| ORCA 4E IBIS file
[IBIS ver]   2.1
[File name]   t_all4e.ibs
[File Rev]   1.3
[Date]   07-29-2004
[Source]   Simulation
[Notes]   IBIS model for ORCA I/O
   These models are non-monotonic to more accurately reflect
   device function. The user should use appropriate IBIS
   simulation techniques.
[Disclaimer] The data in this model is derived from simulations using
   modeling information extracted from the target process. While
   a great deal of care has been taken to provide information
   that is accurate, this model is considered preliminary as it
   has not been verified by actual silicon measurement.Treat the
   data in this model as preliminary until actual silicon
   verification is performed.
[Copyright]   None
|   Component t_all4e
[Component]   t_all4e
[Manufacturer]   Lattice Semiconductor
[Package]
| variable   typ   min   max
| Package BA 352
R_pkg   0.3000   0.2600   0.3300
L_pkg   12.0000nH   10.0000nH   14.0000nH
C_pkg   2.0000pF   1.5000pF   2.5000pF
| Package BC432
|R_pkg   0.4100   0.3400   0.4700
|L_pkg   7.5000nH   6.5000nH   9.5000nH
|C_pkg   1.3000pF   1.1500pF   1.8000pF
|Package BM680
|R_pkg   0.3000   0.2600   0.3500
|L_pkg   7.0000nH   5.5000nH   9.5000nH
|C_pkg   0.8500pF   0.700pF   1.5000pF
[Pin]  signal_name   model_name   R_pin   L_pin   C_pin
101   OBLTTL6   OBLTTL6
102   IBLTTL   IBLTTL
103   OZLTTL6   OZLTTL6
104   BZLTTL6   BZLTTL6
105   IBLTTLPD   IBLTTLPD
106   OZLTTL6PD   OZLTTL6PD
107   BZLTTL6PD   BZLTTL6PD
108   IBLTTLPU   IBLTTLPU
109   OZLTTL6PU   OZLTTL6PU
110   BZLTTL6PU   BZLTTL6PU
111   OBLTTL12   OBLTTL12
112   OZLTTL12   OZLTTL12
113   BZLTTL12   BZLTTL12
114   OZLTTL12PD   OZLTTL12PD
115   BZLTTL12PD   BZLTTL12PD
116   OZLTTL12PU   OZLTTL12PU
117   BZLTTL12PU   BZLTTL12PU
118   OBLTTL24   OBLTTL24
119   OZLTTL24   OZLTTL24
120   BZLTTL24   BZLTTL24
121   OZLTTL24PD   OZLTTL24PD
122   BZLTTL24PD   BZLTTL24PD
123   OZLTTL24PU   OZLTTL24PU
124   BZLTTL24PU   BZLTTL24PU
125   OBCMOS186   OBCMOS186
126   IBCMOS18   IBCMOS18
127   OZCMOS186   OZCMOS186
128   BZCMOS186   BZCMOS186
129   IBCMOS18PD   IBCMOS18PD
130   OZCMOS186PD   OZCMOS186PD
131   BZCMOS186PD   BZCMOS186PD
132   IBCMOS18PU   IBCMOS18PU
133   OZCMOS186PU   OZCMOS186PU
134   BZCMOS186PU   BZCMOS186PU
135   OBCMOS1812   OBCMOS1812
136   OZCMOS1812   OZCMOS1812
137   BZCMOS1812   BZCMOS1812
138   OZCMOS1812PD   OZCMOS1812PD
139   BZCMOS1812PD   BZCMOS1812PD
140   OZCMOS1812PU   OZCMOS1812PU
141   BZCMOS1812PU   BZCMOS1812PU
142   OBCMOS1824   OBCMOS1824
143   OZCMOS1824   OZCMOS1824
144   BZCMOS1824   BZCMOS1824
145   OZCMOS1824PD   OZCMOS1824PD
146   BZCMOS1824PD   BZCMOS1824PD
147   OZCMOS1824PU   OZCMOS1824PU
148   BZCMOS1824PU   BZCMOS1824PU
149   OBCMOS26   OBCMOS26
150   IBCMOS2   IBCMOS2
151   OZCMOS26   OZCMOS26
152   BZCMOS26   BZCMOS26
153   IBCMOS2PD   IBCMOS2PD
154   OZCMOS26PD   OZCMOS26PD
155   BZCMOS26PD   BZCMOS26PD
156   IBCMOS2PU   IBCMOS2PU
157   OZCMOS26PU   OZCMOS26PU
158   BZCMOS26PU   BZCMOS26PU
159   OBCMOS212   OBCMOS212
160   OZCMOS212   OZCMOS212
161   BZCMOS212   BZCMOS212
162   OZCMOS212PD   OZCMOS212PD
163   BZCMOS212PD   BZCMOS212PD
164   OZCMOS212PU   OZCMOS212PU
165   BZCMOS212PU   BZCMOS212PU
166   OBCMOS224   OBCMOS224
167   OZCMOS224   OZCMOS224
168   BZCMOS224   BZCMOS224
169   OZCMOS224PD   OZCMOS224PD
170   BZCMOS224PD   BZCMOS224PD
171   OZCMOS224PU   OZCMOS224PU
172   BZCMOS224PU   BZCMOS224PU
173   OBGTL   OBGTL
174   IBGTL   IBGTL
175   OZGTL   OZGTL
176   BZGTL   BZGTL
177   OBGTLP   OBGTLP
178   IBGTLP   IBGTLP
179   OZGTLP   OZGTLP
180   BZGTLP   BZGTLP
181   OBHSTL   OBHSTL
182   IBHSTL   IBHSTL
183   OZHSTL   OZHSTL
184   BZHSTL   BZHSTL
185   OBPCI   OBPCI
186   IBPCI   IBPCI
187   OZPCI   OZPCI
188   BZPCI   BZPCI
189   OBPECL   OBPECL
190   IBPECL   IBPECL
191   OBSSTL3   OBSSTL3
192   IBSSTL3   IBSSTL3
193   OZSSTL3   OZSSTL3
194   BZSSTL3   BZSSTL3
195   OBSSTL2   OBSSTL2
196   IBSSTL2   IBSSTL2
197   OZSSTL2   OZSSTL2
198   BZSSTL2   BZSSTL2
203   OBLTTL6F   OBLTTL6F
204   OZLTTL6F   OZLTTL6F
205   BZLTTL6F   BZLTTL6F
206   OZLTTL6FPD   OZLTTL6FPD
207   BZLTTL6FPD   BZLTTL6FPD
208   OZLTTL6FPU   OZLTTL6FPU
209   BZLTTL6FPU   BZLTTL6FPU
210   OBLTTL12F   OBLTTL12F
211   OZLTTL12F   OZLTTL12F
212   BZLTTL12F   BZLTTL12F
213   OZLTTL12FPD   OZLTTL12FPD
214   BZLTTL12FPD   BZLTTL12FPD
215   OZLTTL12FPU   OZLTTL12FPU
216   BZLTTL12FPU   BZLTTL12FPU
217   OBLTTL24F   OBLTTL24F
218   OZLTTL24F   OZLTTL24F
219   BZLTTL24F   BZLTTL24F
220   OZLTTL24FPD   OZLTTL24FPD
221   BZLTTL24FPD   BZLTTL24FPD
222   OZLTTL24FPU   OZLTTL24FPU
223   BZLTTL24FPU   BZLTTL24FPU
224   OBCMOS186F   OBCMOS186F
225   OZCMOS186F   OZCMOS186F
226   BZCMOS186F   BZCMOS186F
227   OZCMOS186FPD   OZCMOS186FPD
228   BZCMOS186FPD   BZCMOS186FPD
229   OZCMOS186FPU   OZCMOS186FPU
230   BZCMOS186FPU   BZCMOS186FPU
231   OBCMOS1812F   OBCMOS1812F
232   OZCMOS1812F   OZCMOS1812F
233   BZCMOS1812F   BZCMOS1812F
234   OZCMOS1812FPD  OZCMOS1812FPD
235   BZCMOS1812FPD  BZCMOS1812FPD
236   OZCMOS1812FPU  OZCMOS1812FPU
237   BZCMOS1812FPU  BZCMOS1812FPU
238   OBCMOS1824F   OBCMOS1824F
239   OZCMOS1824F   OZCMOS1824F
240   BZCMOS1824F   BZCMOS1824F
241   OZCMOS1824FPD  OZCMOS1824FPD
242   BZCMOS1824FPD  BZCMOS1824FPD
243   OZCMOS1824FPU  OZCMOS1824FPU
244   BZCMOS1824FPU  BZCMOS1824FPU
245   OBCMOS26F   OBCMOS26F
246   OZCMOS26F   OZCMOS26F
247   BZCMOS26F   BZCMOS26F
248   OZCMOS26FPD   OZCMOS26FPD
249   BZCMOS26FPD   BZCMOS26FPD
250   OZCMOS26FPU   OZCMOS26FPU
251   BZCMOS26FPU   BZCMOS26FPU
252   OBCMOS212F   OBCMOS212F
253   OZCMOS212F   OZCMOS212F
254   BZCMOS212F   BZCMOS212F
255   OZCMOS212FPD   OZCMOS212FPD
256   BZCMOS212FPD   BZCMOS212FPD
257   OZCMOS212FPU   OZCMOS212FPU
258   BZCMOS212FPU   BZCMOS212FPU
259   OBCMOS224F   OBCMOS224F
260   OZCMOS224F   OZCMOS224F
261   BZCMOS224F   BZCMOS224F
262   OZCMOS224FPD   OZCMOS224FPD
263   BZCMOS224FPD   BZCMOS224FPD
264   OZCMOS224FPU   OZCMOS224FPU
265   BZCMOS224FPU   BZCMOS224FPU
266   OBHSTL18   OBHSTL18
267   IBHSTL18   IBHSTL18
268   OZHSTL18   OZHSTL18
269   BZHSTL18   BZHSTL18
301p   OBLVDSp   OBLVDS
301n   OBLVDSn   OBLVDS
302p   IBLVDSp   IBLVDS
302n   IBLVDSn   IBLVDS
303p   OBLVPECLp   OBLVPECL
303n   OBLVPECLn   OBLVPECL
304p   IBLVPECLp   IBLVPECL
304n   IBLVPECLn   IBLVPECL
305p   OBLVDSEp   OBLVDSE
305n   OBLVDSEn   OBLVDSE
306p   IBLVDSEp   IBLVDSE
306n   IBLVDSEn   IBLVDSE
[Diff pin] inv_pin  vdiff  tdelay_typ tdelay_min tdelay_max
301p   301n   0V   0ns   0ns   0ns| Output pin Pair
302p   302n   400mV   0ns   0ns   0ns| Input pin Pair
303p   303n   0V   0ns   0ns   0ns| Output pin Pair
304p   304n   750mV   0ns   0ns   0ns| Input pin Pair
| Models and submodels in the file (171): OBLTTL6 (Output), IBLTTL (Input), OZLTTL6 (3-state), BZLTTL6 (I/O), IBLTTLPD (Input), OZLTTL6PD (3-state), BZLTTL6PD (I/O), IBLTTLPU (Input), OZLTTL6PU (3-state), BZLTTL6PU (I/O), OBLTTL12 (Output), OZLTTL12 (3-state), BZLTTL12 (I/O), OZLTTL12PD (3-state), BZLTTL12PD (I/O), OZLTTL12PU (3-state), BZLTTL12PU (I/O), OBLTTL24 (Output), OZLTTL24 (3-state), BZLTTL24 (I/O), OZLTTL24PD (3-state), BZLTTL24PD (I/O), OZLTTL24PU (3-state), BZLTTL24PU (I/O), OBCMOS186 (Output), IBCMOS18 (Input), OZCMOS186 (3-state), BZCMOS186 (I/O), IBCMOS18PD (Input), OZCMOS186PD (3-state), BZCMOS186PD (I/O), IBCMOS18PU (Input), OZCMOS186PU (3-state), BZCMOS186PU (I/O), OBCMOS1812 (Output), OZCMOS1812 (3-state), BZCMOS1812 (I/O), OZCMOS1812PD (3-state), BZCMOS1812PD (I/O), OZCMOS1812PU (3-state), BZCMOS1812PU (I/O), OBCMOS1824 (Output), OZCMOS1824 (3-state), BZCMOS1824 (I/O), OZCMOS1824PD (3-state), BZCMOS1824PD (I/O), OZCMOS1824PU (3-state), BZCMOS1824PU (I/O), OBCMOS26 (Output), IBCMOS2 (Input), OZCMOS26 (3-state), BZCMOS26 (I/O), IBCMOS2PD (Input), OZCMOS26PD (3-state), BZCMOS26PD (I/O), IBCMOS2PU (Input), OZCMOS26PU (3-state), BZCMOS26PU (I/O), OBCMOS212 (Output), OZCMOS212 (3-state), BZCMOS212 (I/O), OZCMOS212PD (3-state), BZCMOS212PD (I/O), OZCMOS212PU (3-state), BZCMOS212PU (I/O), OBCMOS224 (Output), OZCMOS224 (3-state), BZCMOS224 (I/O), OZCMOS224PD (3-state), BZCMOS224PD (I/O), OZCMOS224PU (3-state), BZCMOS224PU (I/O), OBGTL (Output), IBGTL (Input), OZGTL (3-state), BZGTL (I/O), OBGTLP (Output), IBGTLP (Input), OZGTLP (3-state), BZGTLP (I/O)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
